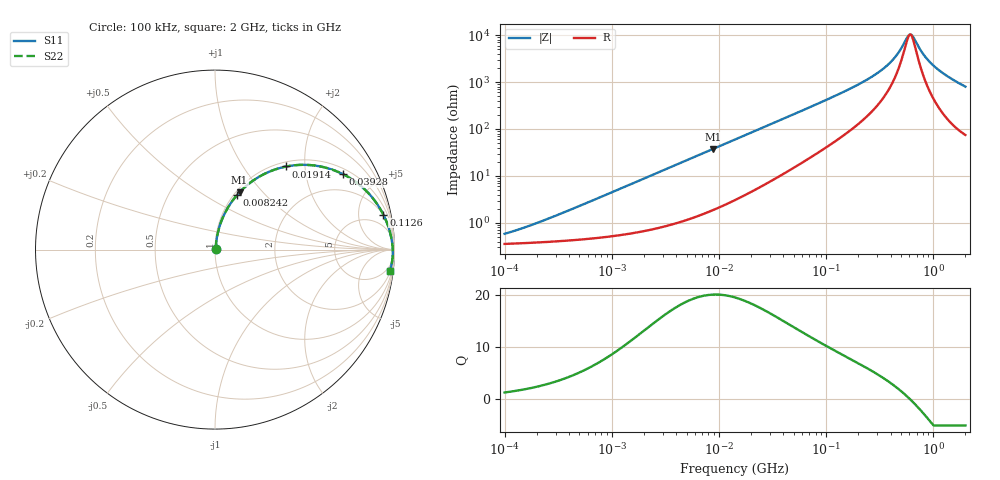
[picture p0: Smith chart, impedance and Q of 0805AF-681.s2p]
# MHz  S  MA  R  50
!Freq  MagS11  AngS11  MagS21  AngS21  MagS12  AngS12  MagS22  AngS22
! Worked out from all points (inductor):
!   801 points, 100 kHz to 2 GHz, reference 50 ohm
!   read as one part in series: L = 724 nH near 259.7 kHz
!   highest Q = 20 at 8.879 MHz (marker M1), where L = 677 nH
!   self-resonance near 607.7 MHz
!   S11 on the Smith chart (normalised r, x): 100 kHz: 1.01, +0.01; 8.242 MHz: 1.04, +0.70; 19.14 MHz: 1.09, +1.60; 39.28 MHz: 1.22, +3.25; 112.6 MHz: 1.97, +9.33; 2 GHz: 2, -16
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0.1  0.005842 52.2  0.9964 -0.3  0.9964 -0.3  0.005842 52.2
0.1928656  0.009607 66.2  0.9962 -0.5  0.9962 -0.5  0.009607 66.2
0.5262716  0.02401 78.0  0.9953 -1.4  0.9953 -1.4  0.02401 78.0
2.735506  0.1178 79.5  0.9854 -6.7  0.9854 -6.7  0.1178 79.5
8.242335  0.3267 68.1  0.9289 -19.0  0.9289 -19.0  0.3267 68.1
8.878575  0.3481 66.8  0.9203 -20.3  0.9203 -20.3  0.3481 66.8
14.21888  0.5031 56.9  0.8388 -30.2  0.8388 -30.2  0.5031 56.9
19.14421  0.6101 49.4  0.76 -37.5  0.76 -37.5  0.6101 49.4
27.08557  0.7274 40.1  0.6447 -46.6  0.6447 -46.6  0.7274 40.1
39.28284  0.8277 30.5  0.5089 -55.7  0.5089 -55.7  0.8277 30.5
73.90831  0.9271 17.6  0.3042 -67.5  0.3042 -67.5  0.9271 17.6
112.6385  0.9581 11.7  0.2043 -72.4  0.2043 -72.4  0.9581 11.7
239.8826  0.9817 5.0  0.08799 -75.5  0.08799 -75.5  0.9817 5.0
384.1679  0.9876 2.2  0.04088 -71.3  0.04088 -71.3  0.9876 2.2
468.4202  0.9891 1.3  0.0244 -62.9  0.0244 -62.9  0.9891 1.3
578.2724  0.9902 0.3  0.01074 -24.0  0.01074 -24.0  0.9902 0.3
622.9102  0.9905 -0.1  0.009689 10.1  0.009689 10.1  0.9905 -0.1
662.7294  0.9906 -0.4  0.01159 35.8  0.01159 35.8  0.9906 -0.4
818.1502  0.9908 -1.4  0.0262 68.8  0.0262 68.8  0.9908 -1.4
985.2932  0.9905 -2.4  0.04217 75.8  0.04217 75.8  0.9905 -2.4
1343.135  0.9884 -4.2  0.07294 78.8  0.07294 78.8  0.9884 -4.2
2000  0.981 -7.0  0.1229 77.6  0.1229 77.6  0.981 -7.0
